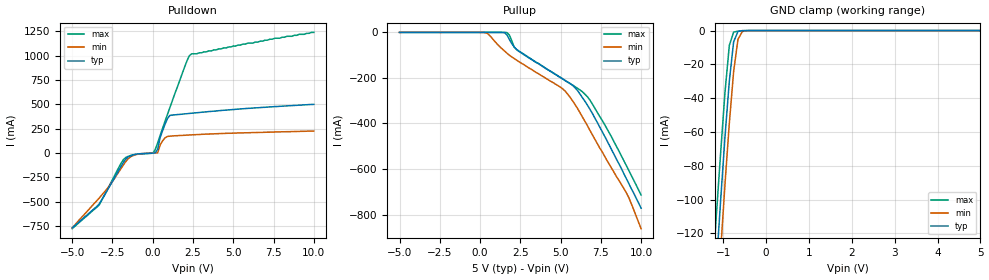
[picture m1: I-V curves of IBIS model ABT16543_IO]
|   TEXAS INSTRUMENTS INCORPORATED
|   Advanced Bus Interface Group
|   IBIS Model of SN74ABT16543
|   16-BIT REGISTERED TRANSCEIVERS WITH 3-STATE OUTPUTS
|   56-pin DL, DGG Package
[IBIS Ver]   2.1
[Comment char]  |_char
[File Name]   abt16543.ibs
[File Rev]   2.0
[Date]   04/15/96
[Source]   File originated at Texas Instruments Incorporated.
[Notes]   The following is a sample IBIS file for the ABT16543.
   - This file may be incomplete or may not be fully compliant
   with the IBIS specification. It will be replaced with a
   version that is IBIS Revision 3.2 compliant and is complete
   and accurate. Please email all questions and comments to
   sllibis@ti.com.
|   - All test data contained in this file are derived from
|   hspice(tm) simulations.
|   - File created by Tareq Shahwan, ABL Applications
|   - Disclaimer modified by David Holmgreen, Launch Marketing
[Disclaimer] Property of Texas Instruments Incorporated.  Unauthorized
   reproduction and/or distribution is strictly prohibited.
   This product is protected under copyright law.
   Created 1995, (C) Copyright 1995, Texas Instruments
   Incorporated, All Rights Reserved
   UNLESS THERE IS A SIGNED, WRITTEN AGREEMENT TO THE
   CONTRARY, TEXAS INSTRUMENTS ("TI") IS PROVIDING THE IBIS
   MODELS "AS IS" AND WITHOUT ANY WARRANTY, EXPRESSED OR
   IMPLIED.  TI assumes no liability for:
   1) the accuracy of the IBIS models provided to your
   company;
   2) the proper functioning of these IBIS models in your
   design or for any resulting applications; or
   3) infringement of patents, copyrights or intellectual
   property rights resulting from your use of these IBIS
   models.
   TI provides IBIS Models as a service to our customers.
   You and your company shall not distribute, sell or give
   these models to anyone else without prior written
   permission from TI.
   TI reserves the right to make changes to our products or
   to discontinue any semiconductor product or service
   without notice, and advises our customers to obtain the
   latest version of relevant information to verify, before
   placing orders, that the information being relied on is
   current.
   Please be aware that your receipt and use of the IBIS
   information provided shall serve as acceptance of these
   terms and conditions.  If you do not accept these terms,
   you should return or destroy the IBIS models and any
   other accompanying information immediately.
[Component]   ABT16543_DGG
[manufacturer]   Texas Instruments Incorporated
[Package]
|   typ   min   max
   R_pkg   0.045   0.035   0.062
   L_pkg   3.324nH   2.403nH   5.094nH
   C_pkg   0.564pF   0.341pF   0.914nH
[Pin]   signal_name   model_name   R_pin   L_pin   C_pin
1   1OEAB_BAR   NC   0.062   5.094nH   0.856pF
2   1LEAB_BAR   NC   0.061   4.621nH   0.902pF
3   1CEAB_BAR   NC   0.06   4.316nH   0.802pF
4   GND   GND   0.059   3.968nH   0.698pF
5   1A1   ABT16543_IO   0.057   3.716nH   0.649pF
6   1A2   ABT16543_IO   0.042   3.517nH   0.652pF
7   VCC   POWER   0.041   3.16nH   0.57pF
8   1A3   ABT16543_IO   0.039   2.981nH   0.482pF
9   1A4   ABT16543_IO   0.039   2.809nH   0.447pF
10   1A5   ABT16543_IO   0.038   2.715nH   0.409pF
11   GND   GND   0.041   2.675nH   0.391pF
12   1A6   ABT16543_IO   0.039   2.536nH   0.366pF
13   1A7   ABT16543_IO   0.039   2.457nH   0.348pF
14   1A8   ABT16543_IO   0.038   2.411nH   0.353pF
15   2A1   ABT16543_IO   0.039   2.456nH   0.355pF
16   2A2   ABT16543_IO   0.039   2.471nH   0.349pF
17   2A3   ABT16543_IO   0.04   2.58nH   0.37pF
18   GND   GND   0.038   2.651nH   0.389pF
19   2A4   ABT16543_IO   0.038   2.739nH   0.411pF
20   2A5   ABT16543_IO   0.039   2.838nH   0.449pF
21   2A6   ABT16543_IO   0.038   2.988nH   0.484pF
22   VCC   POWER   0.038   3.105nH   0.564pF
23   2A7   ABT16543_IO   0.04   3.427nH   0.638pF
24   2A8   ABT16543_IO   0.056   3.654nH   0.641pF
25   GND   GND   0.057   3.932nH   0.7pF
26   2CEAB_BAR   NC   0.058   4.257nH   0.806pF
27   2LEAB_BAR   NC   0.057   4.58nH   0.914pF
28   2OEAB_BAR   NC   0.059   5.038nH   0.861pF
29   2OEBA_BAR   NC   0.06   5.058nH   0.858pF
30   2LEBA_BAR   NC   0.056   4.543nH   0.904pF
31   2CEBA_BAR   NC   0.057   4.24nH   0.803pF
32   GND   GND   0.057   3.929nH   0.7pF
33   2B8   ABT16543_IO   0.056   3.616nH   0.637pF
34   2B7   ABT16543_IO   0.037   3.368nH   0.64pF
35   VCC   POWER   0.036   3.024nH   0.563pF
36   2B6   ABT16543_IO   0.035   2.876nH   0.474pF
37   2B5   ABT16543_IO   0.035   2.745nH   0.444pF
38   2B4   ABT16543_IO   0.037   2.683nH   0.405pF
39   GND   GND   0.038   2.603nH   0.382pF
40   2B3   ABT16543_IO   0.038   2.51nH   0.362pF
41   2B2   ABT16543_IO   0.036   2.412nH   0.341pF
42   2B1   ABT16543_IO   0.038   2.416nH   0.349pF
43   1B8   ABT16543_IO   0.037   2.403nH   0.349pF
44   1B7   ABT16543_IO   0.037   2.429nH   0.341pF
45   1B6   ABT16543_IO   0.036   2.482nH   0.358pF
46   GND   GND   0.037   2.615nH   0.381pF
47   1B5   ABT16543_IO   0.035   2.669nH   0.402pF
48   1B4   ABT16543_IO   0.036   2.763nH   0.442pF
49   1B3   ABT16543_IO   0.036   2.942nH   0.478pF
50   VCC   POWER   0.035   3.053nH   0.564pF
51   1B2   ABT16543_IO   0.036   3.409nH   0.641pF
52   1B1   ABT16543_IO   0.058   3.698nH   0.641pF
53   GND   GND   0.059   3.975nH   0.697pF
54   1CEBA_BAR   NC   0.061   4.327nH   0.802pF
55   1LEBA_BAR   NC   0.061   4.624nH   0.905pF
56   1OEBA_BAR   NC   0.06   5.063nH   0.858pF
[Component]   ABT16543_DL
[manufacturer]   Texas Instruments Incorporated
[Package]
|   typ   min   max
R_pkg   0.055   0.048   0.067
L_pkg   6.539nH   4.802nH   9.746nH
C_pkg   .857pF   0.5pF   1.351pF
[Pin]   signal_name   model_name   R_pin   L_pin   C_pin
1   1OEAB_BAR   NC   0.064   9.646nH   1.202pF
2   1LEAB_BAR   NC   0.059   8.723nH   1.348pF
3   1CEAB_BAR   NC   0.059   8.139nH   1.223pF
4   GND   GND   0.056   7.554nH   1.088pF
5   1A1   ABT16543_IO   0.054   6.991nH   0.966pF
6   1A2   ABT16543_IO   0.053   6.659nH   0.973pF
7   VCC   POWER   0.055   6.321nH   0.905pF
8   1A3   ABT16543_IO   0.055   5.942nH   0.713pF
9   1A4   ABT16543_IO   0.057   5.767nH   0.678pF
10   1A5   ABT16543_IO   0.054   5.459nH   0.631pF
11   GND   GND   0.051   5.224nH   0.638pF
12   1A6   ABT16543_IO   0.048   5.088nH   0.601pF
13   1A7   ABT16543_IO   0.05   5.021nH   0.518pF
14   1A8   ABT16543_IO   0.051   4.802nH   0.5pF
15   2A1   ABT16543_IO   0.051   4.803nH   0.5pF
16   2A2   ABT16543_IO   0.05   5.021nH   0.518pF
17   2A3   ABT16543_IO   0.048   5.088nH   0.601pF
18   GND   GND   0.051   5.224nH   0.638pF
19   2A4   ABT16543_IO   0.054   5.459nH   0.631pF
20   2A5   ABT16543_IO   0.057   5.768nH   0.677pF
21   2A6   ABT16543_IO   0.055   5.942nH   0.715pF
22   VCC   POWER   0.055   6.321nH   0.907pF
23   2A7   ABT16543_IO   0.053   6.659nH   0.972pF
24   2A8   ABT16543_IO   0.054   6.991nH   0.966pF
25   GND   GND   0.056   7.554nH   1.087pF
26   2CEAB_BAR   NC   0.059   8.139nH   1.223pF
27   2LEAB_BAR   NC   0.059   8.727nH   1.351pF
28   2OEAB_BAR   NC   0.067   9.746nH   1.21pF
29   2OEBA_BAR   NC   0.063   9.63nH   1.203pF
30   2LEBA_BAR   NC   0.06   8.751nH   1.349pF
31   2CEBA_BAR   NC   0.06   8.184nH   1.224pF
32   GND   GND   0.056   7.543nH   1.087pF
33   2B8   ABT16543_IO   0.054   7.005nH   0.969pF
34   2B7   ABT16543_IO   0.056   6.714nH   0.975pF
35   VCC   POWER   0.058   6.384nH   0.909pF
36   2B6   ABT16543_IO   0.057   5.976nH   0.717pF
37   2B5   ABT16543_IO   0.057   5.743nH   0.677pF
38   2B4   ABT16543_IO   0.055   5.469nH   0.631pF
39   GND   GND   0.055   5.328nH   0.644pF
40   2B3   ABT16543_IO   0.052   5.189nH   0.606pF
41   2B2   ABT16543_IO   0.052   5.053nH   0.519pF
42   2B1   ABT16543_IO   0.052   4.825nH   0.502pF
43   1B8   ABT16543_IO   0.054   4.896nH   0.506pF
44   1B7   ABT16543_IO   0.052   5.093nH   0.521pF
45   1B6   ABT16543_IO   0.051   5.179nH   0.608pF
46   GND   GND   0.054   5.314nH   0.645pF
47   1B5   ABT16543_IO   0.055   5.511nH   0.632pF
48   1B4   ABT16543_IO   0.057   5.77nH   0.677pF
49   1B3   ABT16543_IO   0.055   5.956nH   0.716pF
50   VCC   POWER   0.055   6.32nH   0.905pF
51   1B2   ABT16543_IO   0.052   6.621nH   0.968pF
52   1B1   ABT16543_IO   0.053   6.974nH   0.966pF
53   GND   GND   0.057   7.571nH   1.089pF
54   1CEBA_BAR   NC   0.057   8.097nH   1.219pF
55   1LEBA_BAR   NC   0.059   8.723nH   1.349pF
56   1OEBA_BAR   NC   0.061   9.56nH   1.199pF
| Models and submodels in the file (1): ABT16543_IO (I/O)
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|   Model ABT16543_IO
[Model]   ABT16543_IO
Model_type   I/O
Polarity   Inverting
Enable   Active-Low
Vinl = 0.8V
Vinh = 2.0V
|   typ   min   max
C_comp   7.46pF   NA   NA
[Temperature Range]   25   -40   85
[Voltage range]   5.0   4.5   5.5
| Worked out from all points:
|   slope of the pulldown table from 0 to 0.75 V, typ, clamps not added: 2.57 ohm
|   GND clamp passes 1 mA (typ) near -0.67 V on its own axis
[Pullup]
|Voltage   I(typ)   I(min)   I(max)
-5V       7.81nA     7.34nA     6.01nA
303mV     2.92nA     -594uA     2.51nA
1.52V     -1.3mA     -81.6mA    -18.7uA
1.67V     -10.7mA    -91.1mA    -744uA
2.12V     -63.9mA    -115mA     -64.3mA
2.27V     -75.9mA    -122mA     -74.9mA
5.15V     -205mA     -249mA     -205mA
5.91V     -244mA     -318mA     -239mA
6.82V     -337mA     -430mA     -297mA
8.18V     -517mA     -598mA     -461mA
9.09V     -643mA     -705mA     -586mA
10V       -772mA     -862mA     -714mA
[Pulldown]
|Voltage   I(typ)   I(min)   I(max)
-5V       -770mA     -771mA     -778mA
-3.33V    -525mA     -464mA     -535mA
-1.82V    -96.6mA    -122mA     -67.3mA
-1.21V    -20.7mA    -26.7mA    -17.2mA
0V        -1.29mA    -935uA     -2.5mA
303mV     38.5mA     2.72mA     103mA
455mV     157mA      81.1mA     179mA
606mV     227mA      124mA      252mA
909mV     353mA      170mA      395mA
1.06V     386mA      173mA      465mA
2.27V     407mA      185mA      1A
10V       500mA      226mA      1.24A
[GND_Clamp]
|Voltage   I(typ)   I(min)   I(max)
-5V       -2.24A     -2.24A     -2.22A
-1.26V    -180mA     -211mA     -148mA
-1.16V    -139mA     -170mA     -109mA
-1.06V    -100mA     -130mA     -71.9mA
-960mV    -63mA      -91mA      -36.7mA
-859mV    -30mA      -55mA      -8.79mA
-758mV    -6.65mA    -24.2mA    -883uA
-657mV    -509uA     -5.24mA    -366uA
-556mV    -16.6uA    -586uA     -143uA
-455mV    -396nA     -38.8uA    -13.6uA
5V        4.72nA     4.77nA     4.01nA
[Ramp]
|Variable   typ   min   max
dV/dt_r   1.732/0.683n   1.922/0.882n   1.995/0.546n
dV/dt_f   2.781/1.886n   2.992/2.402n   3.117/1.339n
